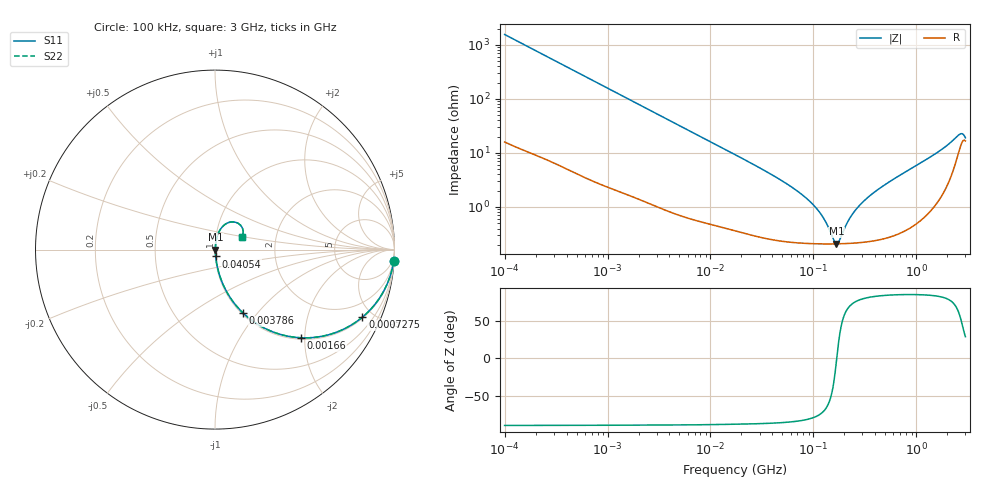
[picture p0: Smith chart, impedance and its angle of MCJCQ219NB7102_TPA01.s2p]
! MCJCQ219NB7102_TPA01  S-PARAMETER MODEL  ( Standard Model )
! Model Generated by TAIYO YUDEN Corporation (http://www.ty-top.com)
! Version 1.0
! TAIYO YUDEN Control No. 220601
! Copyright(c) 2015 TAIYO YUDEN CO.,LTD. All Rights Reserved.
! Product Description (link to TY-COMPAS)
! https://ds.yuden.co.jp/TYCOMPAS/or/detail?pn=MCJCQ219NB7102KTPA01&u=M
! Products Name : Multilayer Ceramic Capacitors
! Characteristics :
!  Capacitance : 1000 [pF] , Rated Voltage : 250 [V] , TCC : X7R
!  Case Size : 2.0 x 1.25 / 0.079 x 0.049 [mm/inch] , Thickness : 0.85 / 0.033 [mm/inch]
!  (Conditions: Temperature = 25 [degC] , DC Bias Voltage = 0 [V])
! External Node Assignments :
!  1  o---| |---o  2
! GND o---------o GND
! Frequency Range : 100kHz  -  3GHz  [ 401 STEP ]
# MHZ S RI R 50
! Freq[MHz].  S11 Real  S11 Imag  S21 Real  S21 Imag  S12 Real  S12 Imag  S22 Real  S22 Imag
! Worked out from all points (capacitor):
!   401 points, 100 kHz to 3 GHz, reference 50 ohm
!   read as one part in series: C = 1.02 nF near 105.3 kHz
!   lowest |Z| = 209 mohm at 167.3 MHz (marker M1)
!   series resonance near 168.6 MHz, so ESL is about 870 pH
!   S11 on the Smith chart (normalised r, x): 100 kHz: 1, -31; 727.5 kHz: 1.06, -4.34; 1.66 MHz: 1.03, -1.91; 3.786 MHz: 1.02, -0.85; 40.54 MHz: 1.00, -0.08; 3 GHz: 1.33, +0.19
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0.1  0.9952 -0.0639  0.00477 0.0639  0.00477 0.0639  0.9952 -0.0639
0.246461  0.974 -0.1531  0.026 0.1531  0.026 0.1531  0.974 -0.1531
0.562235  0.8838 -0.3139  0.1162 0.3139  0.1162 0.3139  0.8838 -0.3139
0.727522  0.8214 -0.3762  0.1786 0.3762  0.1786 0.3762  0.8214 -0.3762
1.659646  0.4787 -0.4912  0.5213 0.4912  0.5213 0.4912  0.4787 -0.4912
3.161081  0.2084 -0.3966  0.7916 0.3966  0.7916 0.3966  0.2084 -0.3966
3.78604  0.1568 -0.3537  0.8432 0.3537  0.8432 0.3537  0.1568 -0.3537
7.027689  0.0547 -0.2152  0.9453 0.2152  0.9453 0.2152  0.0547 -0.2152
17.7727  0.0117 -0.0894  0.9883 0.0894  0.9883 0.0894  0.0117 -0.0894
40.54368  0.00391 -0.0381  0.9961 0.0381  0.9961 0.0381  0.00391 -0.0381
67.88584  0.00259 -0.0203  0.9974 0.0203  0.9974 0.0203  0.00259 -0.0203
97.38194  0.00222 -0.0113  0.9978 0.0113  0.9978 0.0113  0.00222 -0.0113
122.8043  0.00211 -0.0063  0.9979 0.0063  0.9979 0.0063  0.00211 -0.0063
158.9065  0.00207 -0.00116  0.9979 0.00116  0.9979 0.00116  0.00207 -0.00116
167.3121  0.00208 -0.000151  0.9979 0.000151  0.9979 0.000151  0.00208 -0.000151
176.1623  0.00208 0.000858  0.9979 -0.000858  0.9979 -0.000858  0.00208 0.000858
222.1509  0.00215 0.00547  0.9979 -0.00547  0.9979 -0.00547  0.00215 0.00547
273.0175  0.00227 0.00981  0.9977 -0.00981  0.9977 -0.00981  0.00227 0.00981
547.5153  0.00359 0.0289  0.9964 -0.0289  0.9964 -0.0289  0.00359 0.0289
1701.687  0.0255 0.1052  0.9745 -0.1052  0.9745 -0.1052  0.0255 0.1052
2504.792  0.1039 0.1541  0.8961 -0.1541  0.8961 -0.1541  0.1039 0.1541
3000  0.1484 0.0678  0.8516 -0.0678  0.8516 -0.0678  0.1484 0.0678
